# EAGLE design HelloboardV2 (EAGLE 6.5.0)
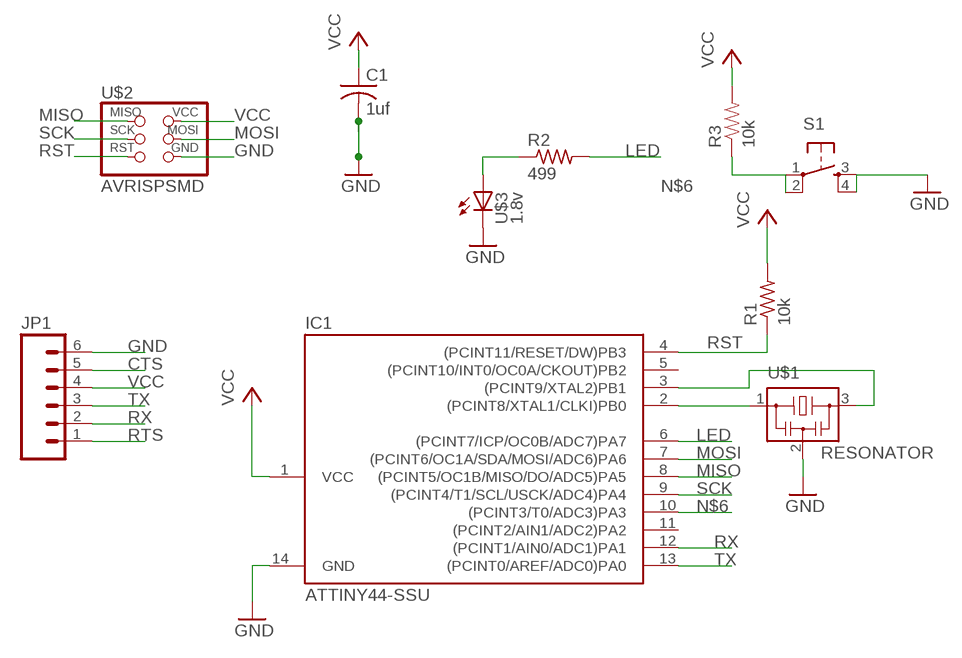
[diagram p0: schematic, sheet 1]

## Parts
C1  1uf  C-USC1206  [C1206]
IC1  ATTINY44-SSU  [SOIC14]
JP1  M06SMD  [1X06-SMD]
R1  10k  R-US_R1206  [R1206]
R2  499  RESISTOR1206  [1206]
R3  10k  RESISTOR  [0805]
S1  6MM_SWITCH6MM_SWITCH  [6MM_SWITCH]
U$1  RESONATOR  [EFOBM]
U$2  AVRISPSMD  [2X03SMD]
U$3  1.8v  LED1206  [1206]

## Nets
CTS: JP1.5
GND: C1.2 IC1.14(GND) JP1.6 S1.3(S) S1.4(S1) U$1.2 U$2.6(GND) U$3.2(C)
LED: IC1.6((PCINT7/ICP/OC0B/ADC7)PA7) R2.2
MISO: IC1.8((PCINT5/OC1B/MISO/DO/ADC5)PA5) U$2.1(MISO)
MOSI: IC1.7((PCINT6/OC1A/SDA/MOSI/ADC6)PA6) U$2.4(MOSI)
N$1: IC1.2((PCINT8/XTAL1/CLKI)PB0) U$1.1
N$2: IC1.3((PCINT9/XTAL2)PB1) U$1.3
N$3: R2.1 U$3.1(A)
N$6: IC1.10((PCINT3/T0/ADC3)PA3) R3.1 S1.1(P) S1.2(P1)
RST: IC1.4((PCINT11/RESET/DW)PB3) R1.1 U$2.5(RST)
RTS: JP1.1
RX: IC1.12((PCINT1/AIN0/ADC1)PA1) JP1.2
SCK: IC1.9((PCINT4/T1/SCL/USCK/ADC4)PA4) U$2.3(SCK)
TX: IC1.13((PCINT0/AREF/ADC0)PA0) JP1.3
VCC: C1.1 IC1.1(VCC) JP1.4 R1.2 R3.2 U$2.2(VCC)
Unconnected: IC1.5((PCINT10/INT0/OC0A/CKOUT)PB2) IC1.11((PCINT2/AIN1/ADC2)PA2)

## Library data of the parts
C1 = rcl:C-US: CAPACITOR, American symbol
IC1 = fab:ATTINY44
JP1 = SparkFun:M06: Header 6 Standard 6-pin 0.1" header. Use with straight break away headers (SKU : PRT-00116), right angle break away headers (PRT-00553), swiss pins (PRT-00743), machine pins (PRT-00117), and female headers (PRT-00115). Molex polarized connector foot print use with SKU : PRT-08094 with associated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
R1 = resistor:R-US_: RESISTOR, American symbol
R2 = ng:RESISTOR
R3 = 01_SparkFun:RESISTOR: Resistor
S1 = ng:6MM_SWITCH: OMRON SWITCH
U$1 = fab:RESONATOR
U$2 = fab:AVRISP
U$3 = ng:LED

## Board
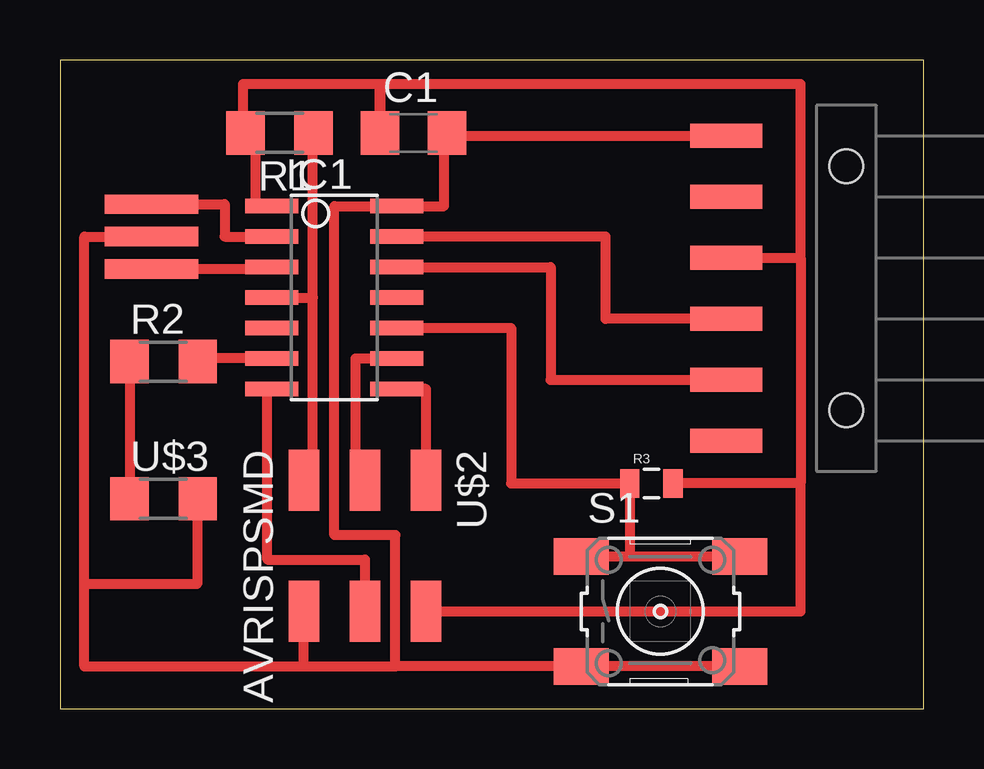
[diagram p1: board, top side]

Size 35.99 x 27.04 mm. Coordinates in mm from the lower left corner, seen from the top.
Outline: 0,0 35.99,0 35.99,27.04 0,27.04 0,0
Copper layers 1: Top 0.035mm
Design rules "ERP-1sided-10mil-16mill": minimum track width 10mil, minimum drill 24mil, track to track 16mil, track to pad 16mil, pad to pad 16mil, via to via 16mil, smd to smd 0mil, copper to edge 16mil, drill to drill 36mil, minimum pad ring 10mil, minimum via ring 8mil, stop-mask expansion 4mil, vias tented up to drill 0mil, thermal gap 10mil

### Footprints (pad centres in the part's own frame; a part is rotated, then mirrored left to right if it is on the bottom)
C1206 = smd 1.6 x 1.8: 1 -1.4,0; 2 1.4,0
SOIC14 = smd 0.61 x 2.21: 1 -3.81,-2.603; 2 -2.54,-2.603; 3 -1.27,-2.603; 4 0,-2.603; 5 1.27,-2.603; 6 2.54,-2.603; 7 3.81,-2.603; 8 3.81,2.603; 9 2.54,2.603; 10 1.27,2.603; 11 0,2.603; 12 -1.27,2.603; 13 -2.54,2.603; 14 -3.81,2.603
1X06-SMD = smd 1 x 3: 1 -6.35,5; 2 -3.81,5; 3 -1.27,5; 4 1.27,5; 5 3.81,5; 6 6.35,5 | hole 1.4: -5.08,0; 5.08,0
R1206 = smd 1.6 x 1.803: 1 -1.422,0; 2 1.422,0
1206 = smd 1.6 x 1.803: 1 -1.422,0; 2 1.422,0
0805 = smd 0.8 x 1.2: 1 -0.9,0; 2 0.9,0
6MM_SWITCH = smd 2.286 x 1.524: 1 -3.302,2.286; 2 3.302,2.286; 3 -3.302,-2.286; 4 3.302,-2.286
EFOBM = smd 0.8 x 3.9: 1 -1.35,0; 2 0,0; 3 1.35,0
2X03SMD = smd 2.54 x 1.27: 1 -2.54,2.54; 2 2.92,2.54; 3 -2.54,0; 4 2.92,0; 5 -2.54,-2.54; 6 2.92,-2.54

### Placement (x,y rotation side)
C1  14.73,24 0 top
IC1  11.43,17.14 270 top
JP1  32.77,17.53 90 top
R1  9.14,24 180 top
R2  4.32,14.48 0 top
R3  24.64,9.4 0 top
S1  25.02,4.06 0 top
U$1  3.81,19.68 270 top
U$2  12.7,6.99 270 top
U$3  4.32,8.76 0 top

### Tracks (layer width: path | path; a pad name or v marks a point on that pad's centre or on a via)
GND
  Top 0.406: 13.97,1.78 13.97,7.24 11.43,7.24 11.43,20.95 IC1.14 16,20.95 16,24 C1.2 16,23.88 JP1.6 27,23.88 | 10.16,1.78 13.97,1.78 | U$1.2 1.02,19.68 1.02,5.21 | U$2.6 10.16,1.78 | 1.02,5.21 1.02,1.78 10.16,1.78 | U$3.2 5.71,8.76 5.71,5.21 1.02,5.21 | S1.4 S1.3 13.97,1.78
LED
  Top 0.406: IC1.6 5.74,14.6 R2.2
MISO
  Top 0.406: IC1.8 15.24,13.33 U$2.1
MOSI
  Top 0.406: IC1.7 8.64,13.33 8.64,6.22 12.7,6.22 U$2.4
N$1
  Top 0.406: U$1.1 6.86,21.04 6.86,19.68 IC1.2
N$2
  Top 0.406: U$1.3 8.83,18.34 IC1.3
N$3
  Top 0.406: R2.1 U$3.1
N$6
  Top 0.406: IC1.10 18.8,15.88 18.8,9.4 R3.1 23.75,6.48 23.75,6.35 | 28.32,6.22 S1.2 23.75,6.35 | 23.75,6.35 S1.1
RST
  Top 0.406: R1.1 10.54,24 10.54,17.14 | IC1.4 10.54,17.14 | U$2.5 10.54,9.52 10.54,17.14
RX
  Top 0.406: IC1.12 20.45,18.41 20.45,13.72 JP1.2
SCK
  Top 0.406: U$2.3 12.32,9.52 12.32,14.6 IC1.9
TX
  Top 0.406: JP1.3 22.73,16.26 22.73,19.68 IC1.13
VCC
  Top 0.406: IC1.1 8.13,20.95 8.13,24 R1.2 7.62,24 7.62,26.04 13.33,26.04 C1.1 13.34,26.04 30.86,26.04 30.86,18.8 | JP1.4 30.86,18.8 | 30.86,18.8 30.86,9.4 | 30.86,9.4 R3.2 | U$2.2 30.86,4.07 30.86,9.4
